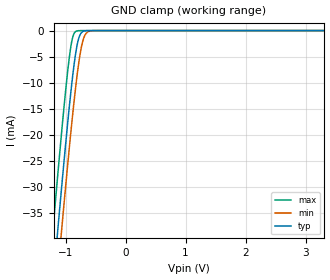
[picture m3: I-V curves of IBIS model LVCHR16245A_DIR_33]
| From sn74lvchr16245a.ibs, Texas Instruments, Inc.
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[Model]   LVCHR16245A_DIR_33
Model_type  Input
Vinl=0.8
Vinh=2.0
| variable   typ   min   max
C_comp   3.50pF   2.64pF   4.72pF
[Temperature Range]   40   100   -40
| Ambient temperature   25   85   -40
[Voltage range]   3.3   3   3.6
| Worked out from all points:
|   GND clamp passes 1 mA (typ) near -0.77 V on its own axis
[GND Clamp]
| LVCHR16245A_DIR_33
|   Voltage   I(typ)   I(min)   I(max)
-5.5V     -655.2mA   -662.2mA   -646.6mA
-1.225V   -50.93mA   -59.21mA   -40.3mA
-1.145V   -40.37mA   -48.66mA   -29.72mA
-1.12V    -37.12mA   -45.41mA   -26.48mA
-1.08V    -31.98mA   -40.25mA   -21.38mA
-1.06V    -29.44mA   -37.69mA   -18.89mA
-965mV    -17.84mA   -25.87mA   -7.89mA
-885mV    -9.098mA   -16.55mA   -1.486mA
-780mV    -1.472mA   -6.227mA   -17.15uA
-715mV    -205.4uA   -2.128mA   -808.5nA
-640mV    -15.53uA   -338.1uA   -23.69nA
3.3V      6.304pA    9.258pA    5.93pA
